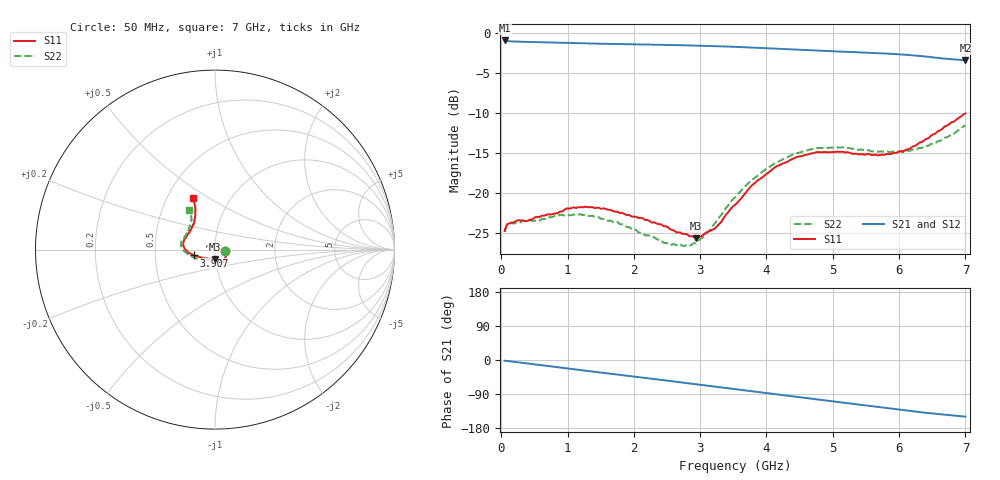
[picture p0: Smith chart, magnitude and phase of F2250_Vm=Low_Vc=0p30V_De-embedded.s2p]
! Integrated Device Technology
! Corporate Headquarters
! 6024 Silver Creek Valley Road
! San Jose, CA 95138  USA
! Phone:  1-408-284-8200
! Toll Free:  1-800-223-1366
! Webpage:  http://www.idt.com/
! Timing and RF Division
! 515 Groton Road, Suite 102
! Westford, MA 01886-6024
! Device:  F2250
! Description: Voltage Variable RF Attenuator
! Frequency:  50.0 -  6000.00 MHz
! Package:  3x3 mm Thin QFN Plastic Package: 16 pin
! Ports:  2 RF, 3 DC
!  Pin  1  = GND
!  Pin  2  = NC
!  Pin  3  = RF1  = Port 1
!  Pin  4  = NC
!  Pin  5  = GND
!  Pin  6  = GND
!  Pin  7  = GND
!  Pin  8  = GND
!  Pin  9  = NC
!  Pin 10  = RF2  = Port 2
!  Pin 11  = NC
!  Pin 12  = GND
!  Pin 13  = GND
!  Pin 14  = VCNTRL
!  Pin 15  = VDD
!  Pin 16  = VMODE
! Vcntrl:  0.300 Volts
! Vmode:  +0.000 Volts
! Vdd:  +3.30  Volts
! Current:  1.115 mA
! Data:  The device was measured on a the F2250 evaluation board which has
!  individual transmission lines to the RF pins.  Data was collected
!  using a calibrated network analyzer.  The evaluation board was
!  de-embedded using a TRL calibration technique.
!  The reference plane is the edge of the package pin.
! Misc:  SN 10
!  Action Tracker AT0258
! Date Measured:  2014-11-26
! Date:  2015-10-15  MJV
! Note:
!  Integrated Device Technology supplies this data as a sample of measured
!  data at the package pin for this product.  Your particular data for this
!  product may vary.
!  Data was taken at 25 degrees C.
!  Integrated Device Technology reserves the right to change this data at anytime.
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# GHz S dB R 50
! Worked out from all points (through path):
!   201 points, 50 MHz to 7 GHz, reference 50 ohm
!   highest |S21| = -0.95 dB at 50 MHz (marker M1); lowest = -3.4 dB at 7 GHz (marker M2)
!   group delay of S21, straight-line fit = 60 ps
!   lowest |S11| = -25.7 dB at 2.934 GHz (marker M3), VSWR 1.11, Z = 49.7 - j5.2 ohm
!   |S11| at or under -10 dB: start of sweep to end of sweep
!   |S22| runs from -26.7 to -11.6 dB; largest |S21 - S12| = 0.00033
!   S11 on the Smith chart (normalised r, x): 50 MHz: 1.12, -0.02; 3.907 GHz: 0.79, -0.05; 7 GHz: 0.67, +0.43
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0.05  -24.74 -9.3  -0.95 -1.8  -0.95 -1.8  -24.87 -9.8
0.08475  -23.93 -9.2  -1.02 -2.5  -1.02 -2.5  -24.00 -9.2
0.15425  -23.71 -11.5  -1.06 -4.0  -1.06 -4.0  -23.76 -10.9
0.57125  -23.03 -29.3  -1.17 -13.1  -1.17 -13.1  -23.49 -30.0
0.884  -22.35 -44.8  -1.23 -19.9  -1.23 -19.9  -22.76 -46.2
1.2315  -21.81 -54.9  -1.31 -27.4  -1.31 -27.4  -22.77 -59.1
1.75275  -22.36 -61.6  -1.40 -38.4  -1.40 -38.4  -23.63 -66.3
2.37825  -23.91 -62.5  -1.49 -51.8  -1.49 -51.8  -25.89 -68.3
2.552  -24.58 -66.6  -1.52 -55.6  -1.51 -55.6  -26.53 -73.9
2.83  -25.38 -81.5  -1.57 -61.7  -1.57 -61.7  -26.64 -92.8
2.93425  -25.65 -90.3  -1.59 -64.0  -1.59 -64.0  -26.29 -101.4
3.21225  -24.50 -119.7  -1.65 -70.2  -1.65 -70.2  -23.90 -127.0
3.525  -21.49 -146.7  -1.75 -77.1  -1.75 -77.1  -20.56 -145.9
3.76825  -19.15 -160.1  -1.84 -82.5  -1.84 -82.5  -18.45 -156.3
3.90725  -18.24 -164.5  -1.89 -85.5  -1.89 -85.5  -17.56 -162.5
4.1505  -16.67 -172.8  -1.99 -90.8  -1.99 -90.8  -16.19 -171.1
4.7065  -15.02 172.9  -2.20 -102.9  -2.20 -102.9  -14.53 175.8
5.15825  -14.88 162.1  -2.36 -112.6  -2.36 -112.6  -14.30 166.6
5.85325  -15.16 138.9  -2.61 -127.5  -2.61 -127.5  -14.91 151.5
6.166  -14.48 128.0  -2.78 -134.3  -2.78 -134.3  -14.73 142.6
6.444  -13.16 119.7  -2.99 -140.1  -2.99 -140.1  -14.12 133.3
7  -10.07 113.3  -3.43 -149.4  -3.43 -149.4  -11.56 123.8
